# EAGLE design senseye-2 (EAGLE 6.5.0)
AUTHOR: Neal Jackson; REV: A; TITLE: SensEye-2
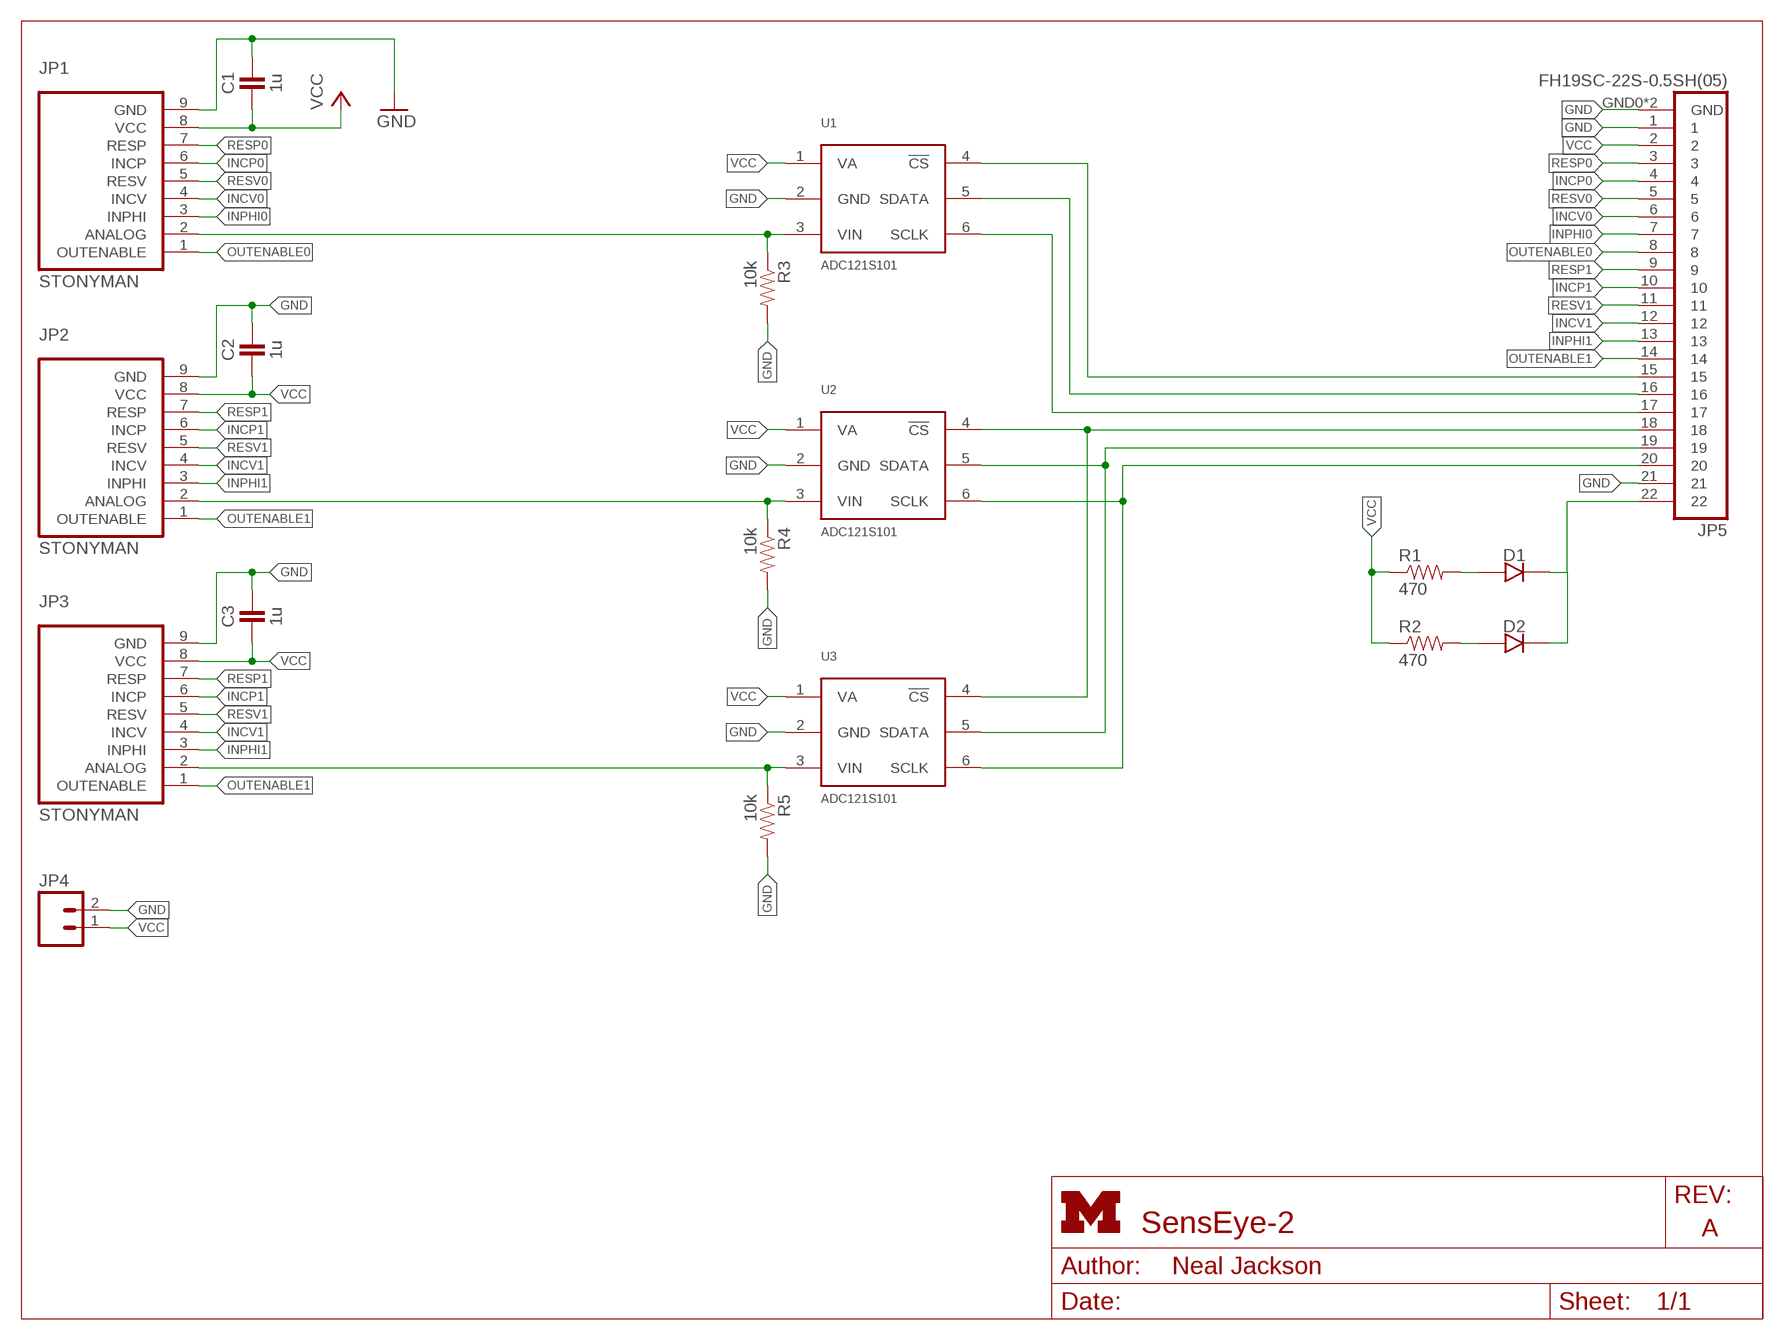
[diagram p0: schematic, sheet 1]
FRAME1 (LETTER_L): HEIGHT: 8.5in; WIDTH: 11in

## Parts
C1  1u  CAPACITOR  [0402_CAP]
C2  1u  CAPACITOR  [0402_CAP]
C3  1u  CAPACITOR  [0402_CAP]
D1  DIODE0603  [0603-DIODE]
D2  DIODE0603  [0603-DIODE]
JP1  STONYMAN  [1X09]
JP2  STONYMAN  [1X09]
JP3  STONYMAN  [1X09]
JP4  M02PTH  [1X02]
JP5  FH19SC-22S-0.5SH(05)  [FH19SC-22S-0.5SH(05)]
R1  470  RESISTOR0402_RES  [0402_RES]
R2  470  RESISTOR0402_RES  [0402_RES]
R3  10k  RESISTOR0402_RES  [0402_RES]
R4  10k  RESISTOR0402_RES  [0402_RES]
R5  10k  RESISTOR0402_RES  [0402_RES]
U1  ADC121S101  [SOT-23-6]
U2  ADC121S101  [SOT-23-6]
U3  ADC121S101  [SOT-23-6]

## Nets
!CS0: JP5.15 U1.4(!CS)
ANALOG0: JP1.2(ANALOG) R3.1 U1.3(VIN)
GND: C1.1 C2.1 C3.1 JP1.9(GND) JP2.9(GND) JP3.9(GND) JP4.2 JP5.1 JP5.21 JP5.GND0(GND) JP5.GND1(GND) R3.2 R4.2 R5.2 U1.2(GND) U2.2(GND) U3.2(GND)
INCP0: JP1.6(INCP) JP5.4
INCP1: JP2.6(INCP) JP3.6(INCP) JP5.10
INCV0: JP1.4(INCV) JP5.6
INCV1: JP2.4(INCV) JP3.4(INCV) JP5.12
INPHI0: JP1.3(INPHI) JP5.7
INPHI1: JP2.3(INPHI) JP3.3(INPHI) JP5.13
LED: D1.2(CATHODE) D2.2(CATHODE) JP5.22
N$1: JP2.2(ANALOG) R4.1 U2.3(VIN)
N$2: D1.1(ANODE) R1.2
N$3: JP3.2(ANALOG) R5.1 U3.3(VIN)
N$5: D2.1(ANODE) R2.2
N$6: JP5.18 U2.4(!CS) U3.4(!CS)
OUTENABLE0: JP1.1(OUTENABLE) JP5.8
OUTENABLE1: JP2.1(OUTENABLE) JP3.1(OUTENABLE) JP5.14
RESP0: JP1.7(RESP) JP5.3
RESP1: JP2.7(RESP) JP3.7(RESP) JP5.9
RESV0: JP1.5(RESV) JP5.5
RESV1: JP2.5(RESV) JP3.5(RESV) JP5.11
SCLK0: JP5.17 U1.6(SCLK)
SCLK1: JP5.20 U2.6(SCLK) U3.6(SCLK)
SDATA0: JP5.16 U1.5(SDATA)
SDATA1: JP5.19 U2.5(SDATA) U3.5(SDATA)
VCC: C1.2 C2.2 C3.2 JP1.8(VCC) JP2.8(VCC) JP3.8(VCC) JP4.1 JP5.2 R1.1 R2.1 U1.1(VA) U2.1(VA) U3.1(VA)

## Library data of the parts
C1-C3 = passives:CAPACITOR: 0402 Capacitor
D1 D2 = passives:DIODE
JP1-JP3 = senseye:STONYMAN: Header 9 Standard 9-pin 0.1" header. Use with straight break away headers (SKU : PRT-00116), right angle break away headers (PRT-00553), swiss pins (PRT-00743), machine pins (PRT-00117), and female headers (PRT-00115).
JP4 = SparkFun-Connectors:M02: Header 2
JP5 = senseye:FH19SC-22S-0.5SH(05)
R1-R5 = passives:RESISTOR: Resistor
U1-U3 = chips:ADC121S101: Analogue to Digital Converter, 12 bit, 1 MSPS, Single, 2.7 V, 5.25 V, SOT-23; DIGIKEY: ADC121S101CIMF/NOPBCT-ND; MOUSER: 926-AD121S101CISDNPB; NEWARK: 96K6188

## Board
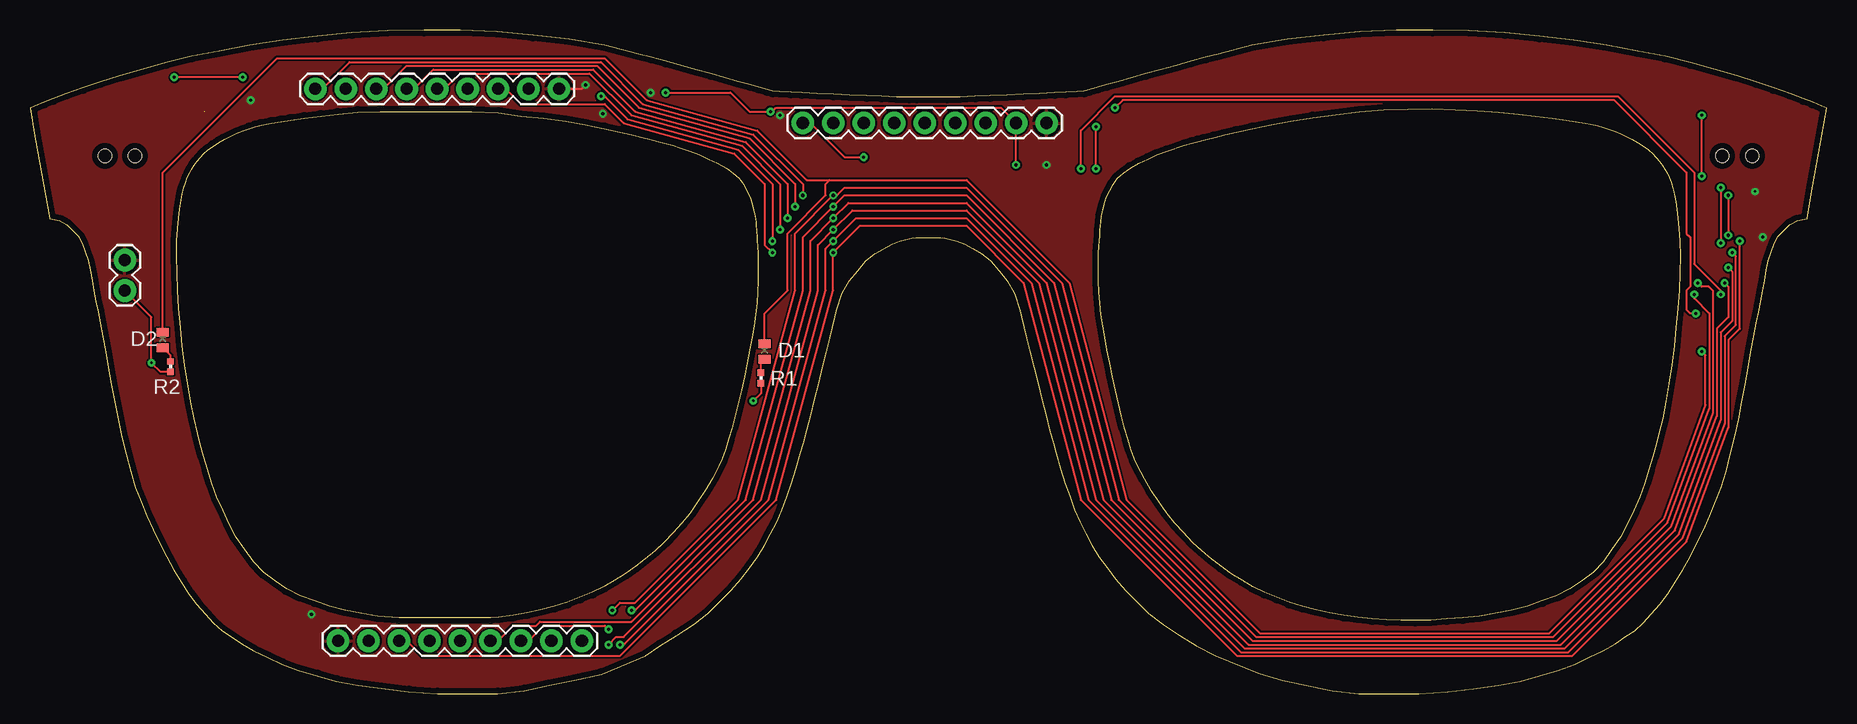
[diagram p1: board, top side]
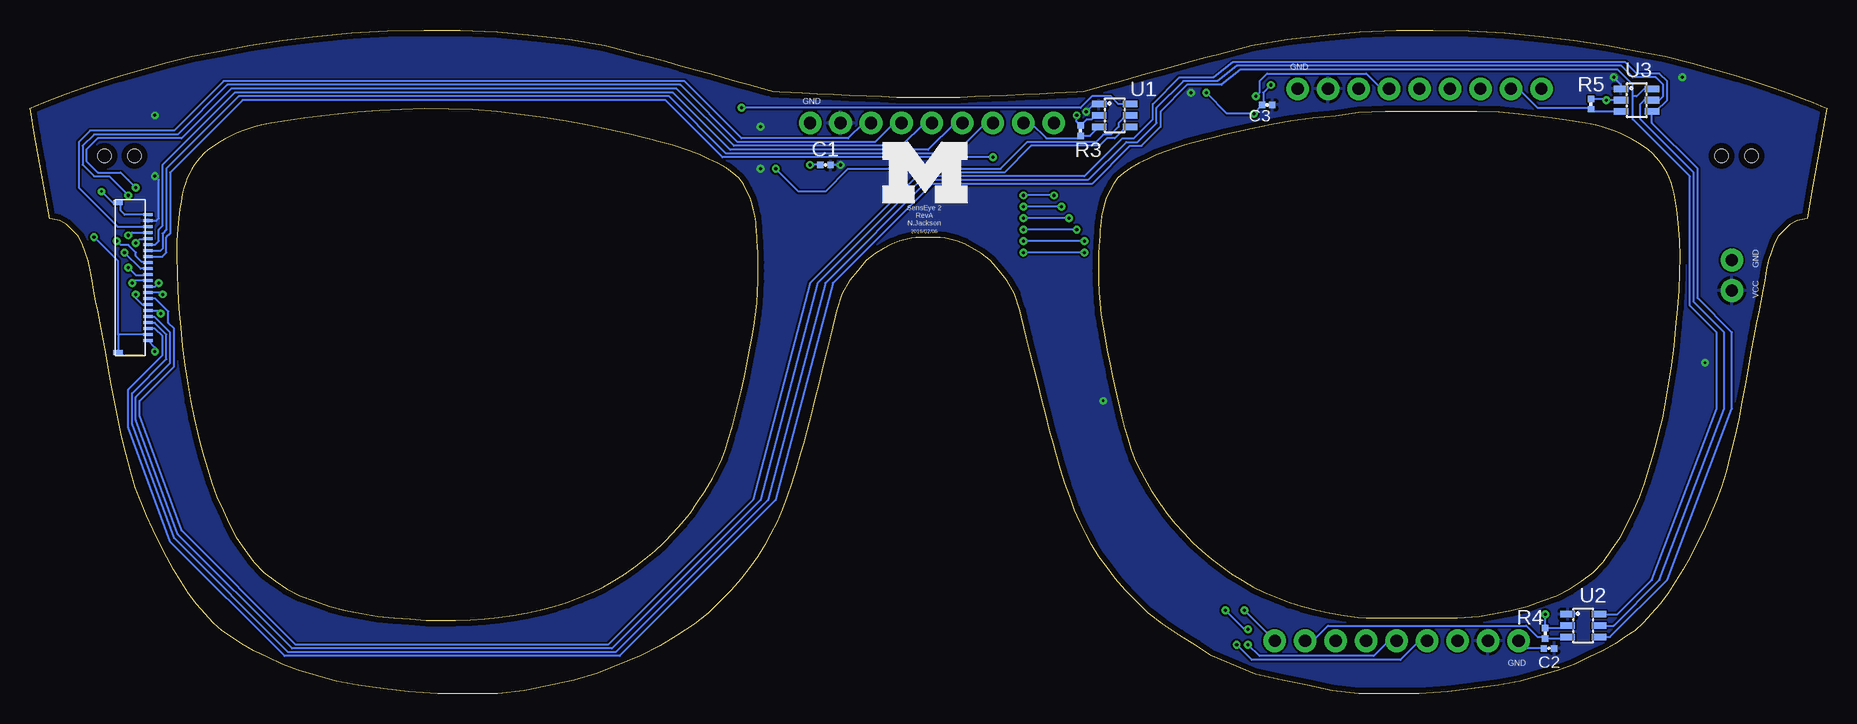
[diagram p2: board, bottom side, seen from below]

Size 149.76 x 55.34 mm. Coordinates in mm from the lower left corner, seen from the top.
Outline: 562 segments
Copper layers (1*16): Top 0.0178mm / dielectric 59mil / Bottom 0.0178mm
Design rules "sunstone-2lyr_v1.0.0.3": minimum track width 6mil, minimum drill 14mil, track to track 6mil, track to pad 6mil, pad to pad 6mil, via to via 6mil, smd to smd 6mil, copper to edge 20mil, drill to drill 16mil, minimum pad ring 8mil, minimum via ring 8mil, stop-mask expansion 3mil, vias tented up to drill 50mil, thermal gap 10mil
Holes 1.1 mm at 6.26,44.83 8.76,44.83 141.06,44.83 143.56,44.83

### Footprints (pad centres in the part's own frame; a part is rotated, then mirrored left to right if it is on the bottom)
0402_CAP = smd 0.536 x 0.546: 1 -0.433,0; 2 0.433,0
0603-DIODE = smd 0.7 x 1: 1 -0.65,0; 2 0.65,0
1X09 = drill 1.016 pad 1.88: 1 0,0; 2 2.54,0; 3 5.08,0; 4 7.62,0; 5 10.16,0; 6 12.7,0; 7 15.24,0; 8 17.78,0; 9 20.32,0
1X02 = drill 1.016 pad 1.88: 1 0,0; 2 2.54,0
FH19SC-22S-0.5SH(05) = smd 0.25 x 0.8: 1 -5.25,0; 2 -4.75,0; 3 -4.25,0; 4 -3.75,0; 5 -3.25,0; 6 -2.75,0; 7 -2.25,0; 8 -1.75,0; 9 -1.25,0; 10 -0.75,0; 11 -0.25,0; 12 0.25,0; 13 0.75,0; 14 1.25,0; 15 1.75,0; 16 2.25,0; 17 2.75,0; 18 3.25,0; 19 3.75,0; 20 4.25,0; 21 4.75,0; 22 5.25,0 | smd 0.4 x 0.8: GND0 -6.25,-2.5; GND1 6.25,-2.5
0402_RES = smd 0.536 x 0.546: 1 -0.433,0; 2 0.433,0
SOT-23-6 = smd 0.55 x 1.2: 1 -0.95,-1.3; 2 0,-1.3; 3 0.95,-1.3; 4 0.95,1.3; 5 0,1.3; 6 -0.95,1.3

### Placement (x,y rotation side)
C1  83.47,44.09 0 bottom
C2  23.14,3.76 0 bottom
C3  46.64,49.09 0 bottom
D1  61.24,28.53 90 top
D2  11.08,29.48 90 top
JP1  64.42,47.58 0 top
JP2  46,4.4 180 top
JP3  23.78,50.44 0 top
JP4  7.9,33.61 90 top
JP5  139.92,34.69 270 bottom
R1  60.92,26.31 90 top
R2  11.71,27.26 90 top
R3  62.19,46.94 90 bottom
R4  23.46,5.03 90 bottom
R5  19.65,49.17 90 bottom
U1  59.34,48.21 270 bottom
U2  20.28,5.67 270 bottom
U3  15.84,49.48 270 bottom
U$1  [UMICH_SOLID_200MIL]  78.7,40.91 0 bottom

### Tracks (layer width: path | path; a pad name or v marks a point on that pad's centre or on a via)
!CS0
  Bottom 0.152: U1.4 58.38,47.26 59.34,46.31 59.97,46.31 60.61,45.67 66.32,45.67 68.54,43.45 75.53,43.45 84.74,34.24 89.5,16.15 101.56,4.08 127.6,4.08 137.12,13.61 140.62,23.13 140.62,24.4 137.76,27.26 137.76,30.43 138.24,30.91 138.24,31.86 139.31,32.94 JP5.15
ANALOG0
  Bottom 0.152: JP1.2 66.32,47.58 65.05,46.31 62.4,46.31 R3.1 61.39,46.51 U1.3
GND  (via drill 0.2, 0.25)
  Top 0.152: JP3.9 46,50.44 v46.32,50.75
  Bottom 0.152: 142.2,40.72 142.2,40.28 141.87,39.94 JP5.1 139.98,40 | 142.2,40.72 JP5.GND0 | v23.46,6.62 R4.2 21.79,5.47 U2.2 | C2.1 25.05,3.76 JP2.9 | U3.2 v18.38,49.48 18.5,49.6 R5.2 | v46.32,50.75 46.95,50.12 46.95,49.2 C3.1 47.07,49.05 v47.75,48.37 49.97,48.37 v51.72,50.12 | v62.51,48.21 62.51,47.69 R3.2 61.68,47.9 61.24,47.9 60.92,48.21 U1.2 | C1.1 v84.74,44.09 | 142.42,29.94 142.42,36.05 v144.43,38.05 | JP5.21 142.42,29.94 | 142.42,29.94 JP5.GND1 | 142.2,40.72 142.2,40.91 142.84,40.91 v143.79,41.86
  pour Top: -0.04,55.83 150.78,55.83 150.78,-0.05 -0.04,-0.05
INCP0  (via drill 0.25)
  Top 0.152: v141.57,41.55 v141.57,38.21
  Bottom 0.152: JP1.6 77.75,47.58 79.34,45.99 90.77,45.99 95.53,50.75 133.31,50.75 137.44,46.63 144.43,46.63 145.38,45.67 145.38,44.09 144.43,43.13 143.16,43.13 v141.57,41.55 | v141.57,38.21 141.49,38.21 141.25,38.45 139.93,38.45 JP5.4
INCP1  (via drill 0.25)
  Top 0.152: v49.18,4.08 49.49,4.08 61.56,16.15 66.32,33.61 66.32,37.1 v66.96,37.74 68.86,39.64 78.07,39.64 83.47,34.24 88.23,16.15 100.93,3.45 128.23,3.45 137.76,12.97 141.25,22.5 141.25,29.8 142.2,30.75 142.2,36.47 v141.89,36.78 | v61.88,37.74 61.88,42.5 59.02,45.36 49.81,47.9 47.91,49.8 v47.59,49.8
  Bottom 0.152: JP2.6 33.94,4.4 35.52,2.81 47.91,2.81 v49.18,4.08 | v61.88,37.74 v66.96,37.74 | JP3.6 37.11,50.44 38.38,51.71 46.64,51.71 47.27,51.07 47.27,50.12 v47.59,49.8 | JP5.10 140.54,35.44 v141.89,36.78
INCV0
  Bottom 0.152: JP1.4 72.67,47.58 74.89,45.36 91.4,45.36 96.17,50.12 132.68,50.12 138.71,44.09 138.71,39.01 139.03,38.69 139.03,37.74 139.33,37.44 JP5.6
INCV1  (via drill 0.25)
  Top 0.152: JP3.4 32.03,50.44 33.62,52.02 46.95,52.02 50.45,48.53 59.65,45.99 63.15,42.5 v63.15,39.64 | JP2.4 39.02,4.4 40.29,5.67 42.19,5.67 42.51,5.99 50.13,5.99 60.29,16.15 65.05,33.61 65.05,37.74 v66.96,39.64 68.23,40.91 78.07,40.91 84.74,34.24 89.5,16.15 101.56,4.08 127.6,4.08 137.12,13.61 140.62,23.13 140.62,30.43 141.57,31.39 141.57,33.93 v141.25,34.24
  Bottom 0.152: v63.15,39.64 v66.96,39.64 | JP5.12 141.06,34.44 v141.25,34.24
INPHI0
  Bottom 0.152: JP1.3 70.13,47.58 72.67,45.04 91.72,45.04 96.48,49.8 132.36,49.8 138.39,43.77 138.39,38.69 138.71,38.37 138.71,37.1 138.87,36.94 JP5.7
INPHI1  (via drill 0.25)
  Top 0.152: JP3.3 29.49,50.44 31.4,52.34 47.27,52.34 50.76,48.85 59.97,46.31 63.78,42.5 v63.78,40.59 | JP2.3 41.56,4.4 42.83,5.67 47.91,5.67 v48.22,5.35 | v50.13,6.94 50.45,6.94 59.65,16.15 64.42,33.61 64.42,38.05 v66.96,40.59 67.91,41.55 78.07,41.55 85.37,34.24 90.13,16.15 101.88,4.4 127.28,4.4 136.81,13.92 140.3,23.45 140.3,33.56 JP5.13 139.33,33.94 v139.03,34.24
  Bottom 0.152: v48.22,5.35 48.54,5.35 v50.13,6.94 | v63.78,40.59 v66.96,40.59 | 139.91,33.93 JP5.13 139.33,33.94 v139.03,34.24
LED  (via drill 0.25)
  Top 0.152: D2.2 11.08,43.45 20.6,52.98 47.91,52.98 51.4,49.48 60.61,46.94 64.73,42.82 66.64,42.82 | D1.2 61.24,31.7 63.15,33.61 63.15,38.37 66.32,41.55 66.32,42.5 66.64,42.82 | 66.64,42.82 78.07,42.82 86.64,34.24 91.4,16.15 102.52,5.03 126.65,5.03 136.17,14.56 139.66,24.08 139.66,28.21 v139.35,28.53
  Bottom 0.152: v139.35,28.53 139.35,28.87 JP5.22
N$1
  Bottom 0.152: JP2.2 42.83,4.4 41.56,5.67 25.05,5.67 24.09,4.72 23.58,4.72 R4.1 21.7,4.6 U2.3
N$2
  Top 0.152: R1.2 60.92,27.56 D1.1
N$3
  Bottom 0.152: U3.3 19.45,48.53 R5.1 19.77,48.85 24.09,48.85 25.68,50.44 JP3.2
N$5
  Top 0.152: R2.2 11.71,28.2 D2.1
N$6  (1 unrouted)
  Bottom 0.152: U2.4 18.06,4.72 13.3,9.48 7.9,23.77 7.9,30.12 10.76,32.97 10.76,43.77 14.57,47.58 14.57,48.5 14.28,48.5 13.3,49.48 13.3,51.07 13.93,51.71 15.84,51.71 16.79,52.66 49.49,52.66 51.08,51.39 53.94,51.39 56.16,49.17 56.16,47.9 57.75,46.31 58.7,46.31 61.88,43.13 75.21,43.13 84.1,34.24 88.86,16.15 101.25,3.76 127.92,3.76 137.44,13.29 140.93,22.81 140.93,24.72 138.08,27.58 138.08,30.12 139.35,31.39 139.87,31.39 JP5.18
OUTENABLE0  (via drill 0.25)
  Top 0.152: JP1.1 65.05,47.58 67.91,44.72 v69.5,44.72
  Bottom 0.152: v69.5,44.72 92.04,44.72 96.8,49.48 132.04,49.48 138.08,43.45 138.08,38.37 138.39,38.05 138.39,36.78 138.74,36.44 JP5.8
OUTENABLE1  (via drill 0.25)
  Top 0.152: JP3.1 24.41,50.44 26.63,52.66 47.59,52.66 51.08,49.17 60.29,46.63 64.42,42.5 v64.42,41.55 | v48.54,6.94 49.18,7.57 50.45,7.57 59.02,16.15 63.78,33.61 63.78,38.37 v66.96,41.55 67.27,41.55 67.91,42.18 78.07,42.18 86.01,34.24 90.77,16.15 102.2,4.72 126.96,4.72 136.49,14.24 139.98,23.77 139.98,31.7 138.71,32.97 v138.71,33.29
  Bottom 0.152: JP2.1 v48.54,6.94 | v64.42,41.55 v66.96,41.55 | 139.91,33.45 JP5.14 138.88,33.44 v138.71,33.29
RESP0
  Bottom 0.152: JP1.7 80.29,47.58 81.56,46.31 90.45,46.31 95.21,51.07 133.63,51.07 137.76,46.94 144.74,46.94 145.7,45.99 145.7,42.18 142.45,38.94 JP5.3
RESP1  (via drill 0.25)
  Top 0.152: JP2.7 31.4,4.4 32.67,3.13 49.18,3.13 62.19,16.15 66.96,33.61 v66.96,36.78 69.18,39.01 78.07,39.01 82.83,34.24 87.59,16.15 100.61,3.13 128.55,3.13 138.08,12.65 141.57,22.18 141.57,29.48 142.52,30.43 v142.52,37.74 | JP3.7 39.65,50.44 40.92,49.17 47.91,49.17 49.49,47.58 58.7,45.04 61.24,42.5 61.24,37.42 v61.88,36.78
  Bottom 0.152: v61.88,36.78 v66.96,36.78 | JP5.9 139.97,35.99 140.46,35.99 140.93,36.47 140.93,36.78 141.57,37.42 142.2,37.42 v142.52,37.74
RESV0  (via drill 0.25)
  Top 0.152: v140.93,42.18 v140.93,37.58
  Bottom 0.152: JP1.5 75.21,47.58 77.12,45.67 91.09,45.67 95.85,50.44 133,50.44 137.12,46.31 144.11,46.31 145.06,45.36 145.06,44.4 144.11,43.45 142.2,43.45 v140.93,42.18 141.57,42.82 | v140.93,37.58 140.62,37.89 139.96,37.89 JP5.5
RESV1  (via drill 0.25)
  Top 0.152: JP3.5 34.57,50.44 35.84,51.71 46.64,51.71 50.13,48.21 59.34,45.67 62.51,42.5 v62.51,38.69 | v48.22,4.08 48.86,4.72 49.49,4.72 60.92,16.15 65.69,33.61 65.69,37.42 v66.96,38.69 68.54,40.28 78.07,40.28 84.1,34.24 88.86,16.15 101.25,3.76 127.92,3.76 137.44,13.29 140.93,22.81 140.93,30.12 141.89,31.07 141.89,35.2 v141.57,35.51
  Bottom 0.152: JP2.5 36.48,4.4 37.75,3.13 47.27,3.13 v48.22,4.08 | v62.51,38.69 v66.96,38.69 | JP5.11 139.98,34.88 140.93,34.88 v141.57,35.51
SCLK0  (via drill 0.25)
  Top 0.152: v138.87,31.7 138.39,31.7 138.08,32.02 138.08,33.61 138.39,33.93 138.39,38.05 138.08,38.37 138.08,43.45 132.04,49.48 91.09,49.48 v90.45,48.85
  Bottom 0.152: U1.6 59.02,49.16 59.65,49.8 61.24,49.8 62.19,48.85 v90.45,48.85 | JP5.17 139.11,31.94 v138.87,31.7
SCLK1
  Bottom 0.152: U2.6 17.43,6.62 14.57,9.48 9.17,23.77 9.17,30.12 11.39,32.34 11.39,43.13 16.16,47.9 16.16,49.8 | 16.16,49.8 16.16,50.75 17.43,52.02 48.86,52.02 50.45,50.75 53.3,50.75 55.53,48.53 55.53,47.26 57.11,45.67 58.07,45.67 61.24,42.5 74.58,42.5 82.83,34.24 87.59,16.15 100.61,3.13 128.55,3.13 138.08,12.65 141.57,22.18 141.57,25.35 138.71,28.21 138.71,29.8 139.35,30.43 JP5.20 | U3.6 15.2,50.44 15.84,49.8 16.16,49.8
SDATA0  (via drill 0.25)
  Top 0.152: v140.93,33.29 140.93,33.61 138.71,35.83 138.71,43.45 132.36,49.8 90.45,49.8 87.59,46.94 v87.59,43.77
  Bottom 0.152: U1.5 58.38,48.21 59.02,47.58 59.02,47.26 59.65,46.63 60.29,46.63 60.92,45.99 66.64,45.99 68.86,43.77 81.56,43.77 83.47,41.86 85.69,41.86 v87.59,43.77 | v140.93,33.29 140.93,32.97 140.4,32.44 JP5.16
SDATA1
  Bottom 0.152: U2.5 17.74,5.67 13.93,9.48 8.54,23.77 8.54,30.12 11.08,32.66 11.08,43.45 15.52,47.9 15.52,49.17 15.2,49.48 U3.5 13.93,49.48 13.62,49.8 13.62,50.75 14.25,51.39 16.16,51.39 17.11,52.34 49.18,52.34 50.76,51.07 53.62,51.07 55.84,48.85 55.84,47.58 57.43,45.99 58.38,45.99 61.56,42.82 74.89,42.82 83.47,34.24 88.23,16.15 100.93,3.45 128.23,3.45 137.76,12.97 141.25,22.5 141.25,25.04 138.39,27.89 138.39,29.96 139.35,30.91 139.89,30.91 JP5.19
VCC  (via drill 0.2, 0.25)
  Top 0.152: v17.74,51.39 v12.03,51.39 | v139.35,43.13 v139.35,48.21 | v82.2,44.09 JP1.8 80.93,48.85 62.19,48.85 61.88,48.53 v61.72,48.53 59.97,48.53 58.38,50.12 v52.99,50.12 | v88.86,43.77 v88.86,47.26 | R1.1 60.92,25.04 v60.29,24.4 | R2.1 10.88,26.83 v10.12,27.58 10.12,31.39 JP4.1
  Bottom 0.152: U3.1 17.14,50.78 v17.74,51.39 | U1.1 61.09,49.16 v61.72,48.53 | JP5.2 139.23,39.44 139.03,39.64 139.03,42.82 v139.35,43.13 | C1.2 v82.2,44.09
  pour Bottom: -0.04,55.83 150.78,55.83 150.78,-0.05 -0.04,-0.05

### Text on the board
bNames: GND | GND | RevA | SensEye 2 | N.Jackson | 2016/02/06 | GND | VCC | GND

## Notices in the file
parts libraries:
SparkFun-Connectors: Licensing: CC v3.0 Share-Alike You are welcome to use this library for commercial purposes.
